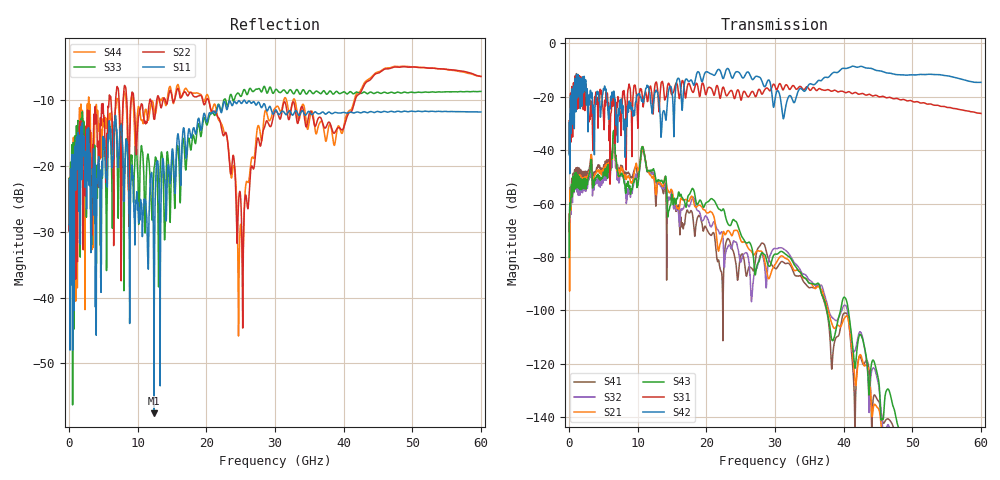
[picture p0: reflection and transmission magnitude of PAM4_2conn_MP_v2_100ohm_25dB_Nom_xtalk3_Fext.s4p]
! Info: Touchstone file created by Circ.  Input file=FAB50GbE_2conn_Midplane_Examax_Topo2_v2_100ohm_25dB_Nom.circ
# Hz S RI R 50
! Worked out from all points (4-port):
!   6000 points, 10 MHz to 60 GHz, reference 50 ohm
!   strongest paths, dB at 10 MHz, 15.01 GHz, 30.01 GHz, 45.01 GHz, 60 GHz:
!     S42: -41.7, -18.2, -20.8, -10.2, -14.6
!     S31: -41.1, -19.1, -16.0, -19.8, -26.2
!     S43: -80.2, -56.5, -78.9, -124.9, -176.7
!     S21: -63.8, -55.1, -82.8, -136.5, -184.5
!     S32: -67.6, -55.3, -76.8, -126.7, -183.4
!     S41: -67.0, -56.8, -84.2, -133.7, -190.1
!   lowest |S11| = -57.6 dB at 12.38 GHz (marker M1), VSWR 1.00, Z = 49.9 + j0.0285 ohm
!   |S11| at or under -10 dB: start of sweep to 25.45 GHz; 25.57 GHz to end of sweep
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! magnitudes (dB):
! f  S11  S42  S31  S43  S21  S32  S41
! 10 MHz  -28.9  -41.7  -41.1  -80.2  -63.8  -67.6  -67.0
! 1.08 GHz  -15.6  -11.5  -11.3  -49.2  -50.3  -54.6  -47.4
! 6.42 GHz  -19.0  -19.1  -21.0  -34.1  -36.5  -38.3  -34.6
! 12.38 GHz  -57.6  -20.7  -19.1  -47.5  -50.0  -48.3  -50.4
! 24.87 GHz  -10.2  -11.1  -19.4  -70.4  -72.6  -80.9  -81.4
! 28.66 GHz  -11.1  -15.7  -16.9  -80.0  -83.8  -89.7  -77.0
! 60 GHz  -11.8  -14.6  -26.2  -176.7  -184.5  -183.4  -190.1
